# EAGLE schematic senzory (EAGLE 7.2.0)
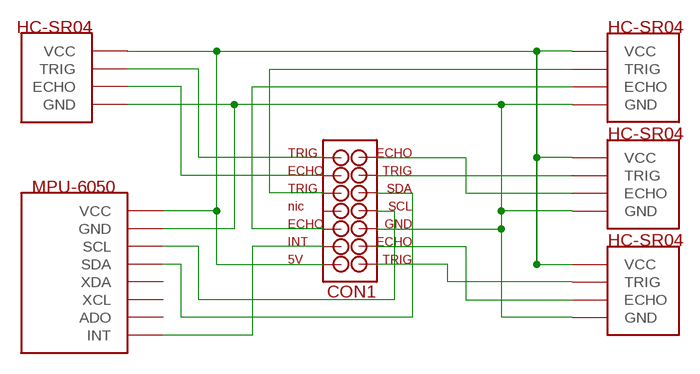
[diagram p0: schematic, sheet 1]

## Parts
U$1  WIFI  [WIFI]
U$2  HC_SR  [CON_4]
U$3  HC_SR  [CON_4]
U$4  HC_SR  [CON_4]
U$5  HC_SR  [CON_4]
U$25  SDA  CON_1  [CON_1]
U$26  INT  CON_1  [CON_1]
U$27  5V  CON_1  [CON_1]
U$28  GND  CON_1  [CON_1]
U$29  ECHO  CON_1  [CON_1]
U$30  TRIG  CON_1  [CON_1]
U$31  ECHO  CON_1  [CON_1]
U$32  TRIG  CON_1  [CON_1]
U$33  SCL  CON_1  [CON_1]
U$34  ECHO  CON_1  [CON_1]
U$35  TRIG  CON_1  [CON_1]
U$36  ECHO  CON_1  [CON_1]
U$37  TRIG  CON_1  [CON_1]
U$38  nic  CON_1  [CON_1]

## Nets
N$2: U$1.P$2(GND) U$2.P$4(GND) U$3.P$4(GND) U$4.P$4(GND) U$5.P$4(GND) U$28.P$1
N$3: U$2.P$2(TRIG) U$30.P$1
N$4: U$2.P$3(ECHO) U$29.P$1
N$5: U$3.P$2(TRIG) U$32.P$1
N$6: U$3.P$3(ECHO) U$31.P$1
N$7: U$4.P$2(TRIG) U$35.P$1
N$8: U$4.P$3(ECHO) U$34.P$1
N$9: U$5.P$2(TRIG) U$37.P$1
N$10: U$5.P$3(ECHO) U$36.P$1
N$11: U$1.P$3(SCL) U$33.P$1
N$12: U$1.P$4(SDA) U$25.P$1
N$13: U$1.P$8(INT) U$26.P$1
N$16: U$1.P$1(VCC) U$2.P$1(VCC) U$3.P$1(VCC) U$4.P$1(VCC) U$5.P$1(VCC) U$27.P$1
Unconnected: U$1.P$5(ADO) U$1.P$6(XCL) U$1.P$7(XDA) U$38.P$1

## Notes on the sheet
- CON1

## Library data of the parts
U$1 = arduino:WIFI
U$2-U$5 = arduino:HC_SR
U$25-U$38 = arduino:CON_1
